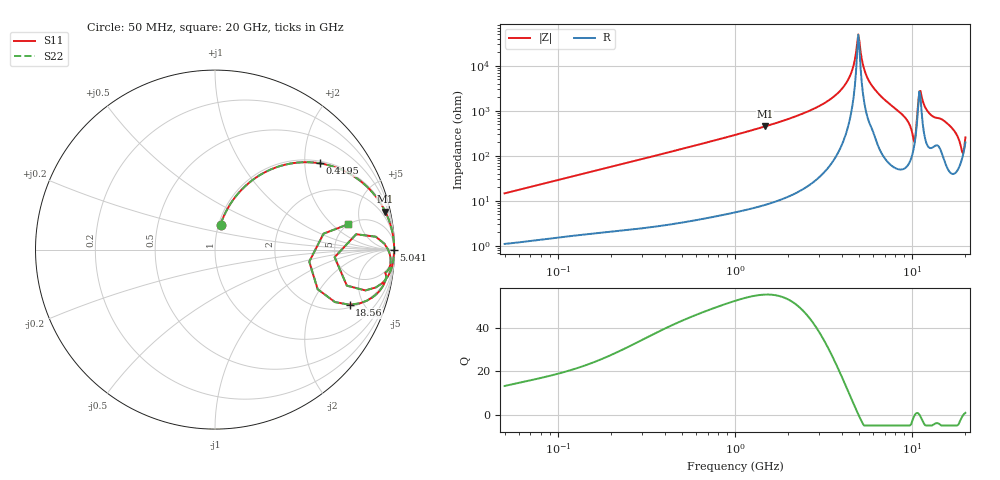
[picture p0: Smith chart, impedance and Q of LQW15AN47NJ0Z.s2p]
!Murata Part Number: LQW15AN47NJ0Z
!These Parameters are Measured in Series Mode Connection
!  o--[Z]--o
!Port1  Port2
!  o-------o
!Freq. Start=50[MHz] Stop=20[GHz], 401[Steps]
# Hz S RI R 50
!Freq.(Hz) S11(Real) S11(Imag) S21(Real) S21(Imag) S12(Real) S12(Imag) S22(Real) S22(Imag)
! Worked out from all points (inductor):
!   401 points, 50 MHz to 20 GHz, reference 50 ohm
!   read as one part in series: L = 46.2 nH near 51.52 MHz
!   highest Q = 55.5 at 1.476 GHz (marker M1), where L = 48.3 nH
!   self-resonance near 4.967 GHz
!   S11 on the Smith chart (normalised r, x): 50 MHz: 1.02, +0.29; 419.5 MHz: 1.06, +2.37; 5.041 GHz: open; 18.56 GHz: 2.19, -3.92; 20 GHz: 4.96, +3.26
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5e7  0.031 0.1397  0.969 -0.1397  0.969 -0.1397  0.031 0.1397
1.364002e8  0.1429 0.3282  0.8571 -0.3282  0.8571 -0.3282  0.1429 0.3282
3.721004e8  0.5251 0.4865  0.4749 -0.4865  0.4749 -0.4865  0.5251 0.4865
4.194704e8  0.583 0.4809  0.417 -0.4809  0.417 -0.4809  0.583 0.4809
1e9  0.8892 0.3045  0.1108 -0.3045  0.1108 -0.3045  0.8892 0.3045
1.476162e9  0.9491 0.2109  0.0509 -0.2109  0.0509 -0.2109  0.9491 0.2109
2.728004e9  0.9892 0.0926  0.0108 -0.0926  0.0108 -0.0926  0.9892 0.0926
4.087748e9  0.9973 0.0296  0.00274 -0.0296  0.00274 -0.0296  0.9973 0.0296
4.472136e9  0.9979 0.0162  0.00214 -0.0162  0.00214 -0.0162  0.9979 0.0162
4.89267e9  0.998 0.00259  0.00197 -0.00259  0.00197 -0.00259  0.998 0.00259
5.041459e9  0.998 -0.00199  0.00202 0.00199  0.00202 0.00199  0.998 -0.00199
5.352748e9  0.9977 -0.0113  0.00233 0.0113  0.00233 0.0113  0.9977 -0.0113
5.683258e9  0.9969 -0.0208  0.00307 0.0208  0.00307 0.0208  0.9969 -0.0208
7.442007e9  0.9919 -0.0691  0.00805 0.0691  0.00805 0.0691  0.9919 -0.0691
9.457416e9  0.9556 -0.16  0.0444 0.16  0.0444 0.16  0.9556 -0.16
1.019291e10  0.7347 -0.201  0.2653 0.201  0.2653 0.201  0.7347 -0.201
1.098561e10  0.964 0.00117  0.036 -0.00117  0.036 -0.00117  0.964 0.00117
1.131968e10  0.977 -0.041  0.023 0.041  0.023 0.041  0.977 -0.041
1.257102e10  0.9681 -0.1086  0.0319 0.1086  0.0319 0.1086  0.9681 -0.1086
1.670968e10  0.9287 -0.214  0.0713 0.214  0.0713 0.214  0.9287 -0.214
1.855685e10  0.75 -0.3072  0.25 0.3072  0.25 0.3072  0.75 -0.3072
2e10  0.7415 0.1412  0.2585 -0.1412  0.2585 -0.1412  0.7415 0.1412
